ORGANIZATION_BLOCK MAIN:OB1
TITLE=Controllo Livello Serbatoio
//Simulatore: 08
//Versione: 1.0
//Data: 28/02/2002
//------------------ Descrizione del Controllo --------------------
// Il selettore SA1 seleziona il modo di funzionamento del controllo;
// in base alla sua impostazione il programma, mediante opportune
// istruzioni di SCR, eseguirà la parte di istruzioni che gestiscono
// i due modi di funzionamento.
// FUNZIONAMENTO IN AUTOMATICO: quando il selettore SA1 viene portato
// nella Posizione "A" il bit SCR S0.0 verrà settato a 1 e il bit
// SCR S0.1 verrà settato a 0. In queste condizioni il programma
// eseguirà solo il primo segmento SCR e salterà il successivo.
// Le condizioni di Start/Stop del funzionamento vengono memorizzate
// nel marker M2.1; lo start del controllo verrà effettuato con il
// pulsante SB2, l'arresto avverrà con l'intervento del pulsante
// SB3 di Stop o con l'intervento del pulsante SB1 che simula
// l'intervento di un'emergenza esterna. Il controllo verrà arrestato
// automaticamente anche in caso di intervento del relè termico del
// motore della pompa P1.
// In automatico viene gestita l'immissione dell'acqua nel serbatoio
// di carico mediante il controllo dell'elettrovalvola YV1 che verrà
// chiusa solamente quando il livello della vasca raggiunge il massimo
// (SL1 a aperto). Il controllo provvede anche ad azionare il motore
// della pompa P1 attraverso il pilotaggio del contattore KM1; la
// pompa sarà sempre in funzione fino a quando il livello del
// serbatoio ha raggiunto il massimo (SL5 aperto) oppure quando il
// livello della vasca di carico scende sotto il minimo (SL2 aperto).
// FUNZIONAMENTO IN MANUALE: in questo modo di funzionamento le
// operazioni precedentemente descritte vengono svolte manualmente
// portando a "1" il selettore SA2 per il carico dell'acqua nella
// vasca e il selettore SA4 per l'azionamento della pompa P1.
// Per le modalità di controllo di YV1 e KM1 valgono le stesse
// considerazioni fatte in precedenza.
// Indipendentemente dal modo di funzionamento è sempre possibile
// effettuare lo scarico del serbatoio agendo sul selettore SA3
// per aprire l'elettrovalvola YV2; nessuna limitazione è prevista
// per questa operazione.
// Le segnalazioni sono affidate a quattro lampade:
// - HL1 Pompa in Funzione
// - HL2 Termico scattato
// - HL3 Vasca di carico sotto il minimo
// - HL4 Modo automatico selezionato
//

BEGIN
NETWORK 1 //Impostazione bit SCR Automatico
//
LD I0.6
= S0.0

NETWORK 2 //Impostazione Bit SCR Manuale
//
LDN I0.6
= S0.1

NETWORK 3 //Inizio Blocco SCR Automatico
//
LSCR S0.0

NETWORK 4 //Start/Stop i modo automatico
//
LD I1.4
O M2.1
A I0.2
A I0.7
A I1.3
= M2.1

NETWORK 5 //Carico Vasca in Automatico
//
LD M2.1
A I0.0
= M0.1

NETWORK 6 //Controllo Pompa P1 in automatico
//
LD M2.1
A I0.1
A I0.5
= M0.0

NETWORK 7 //Fine Blocco SCR Automatico
//
SCRE

NETWORK 8 //Inizio Blocco SCR Manuale
//
LSCR S0.1

NETWORK 9 //Controllo elettrovalvola carico in Manuale
//
//
//
LD I1.0
A I0.0
= M1.1

NETWORK 10 //Controllo Pompa P1 in Manuale (SET)
//
LD I0.1
A I0.5
AN M2.0
A I1.2
= M1.0

NETWORK 11 //Fine Blocco SCR Manuale
//
SCRE

NETWORK 12 //Comando elettrovalvola Scarico serbatoio
//
LD I1.1
= Q0.2

NETWORK 13 //Comando Pompa
//
LD M0.0
O M1.0
= Q0.1

NETWORK 14 //Comando elettrovalvola di carico
//
LD M0.1
O M1.1
= Q0.0

NETWORK 15 //Segnalazione Pompa P1 ON
//
LD Q0.1
= Q0.3

NETWORK 16 //Segnalazione relè termico scattato
//
LDN I0.2
= Q0.4

NETWORK 17 //Segnalazione livello minimo vasca di carico
//
LDN I0.1
= Q0.5

NETWORK 18 //Segnalazione funzionamento in automatico
//
LD I0.6
= Q0.6

NETWORK 19 //merker antiavviamento pompa  manuale (SET)
//
LDN I0.2
S M2.0 1

NETWORK 20 //Merker antiavviamento pompa manuale (RESET)
//
LD I0.2
AN I1.2
EU
R M2.0 1

END_ORGANIZATION_BLOCK

